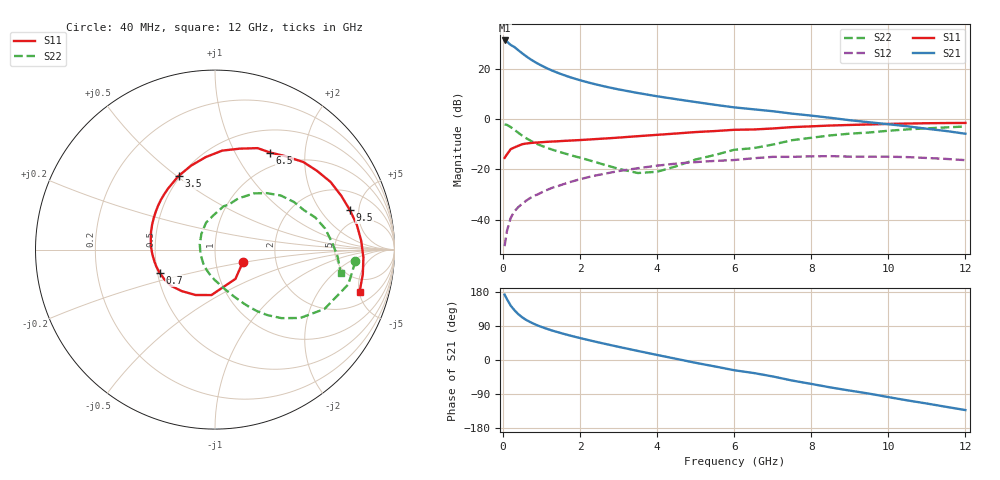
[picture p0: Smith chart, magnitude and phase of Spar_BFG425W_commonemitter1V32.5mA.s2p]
! Filename: 132bfg425.001
! BFG425W Field C1
! V1=8.907E-001V,V2=1.000E+000V, I1=5.288E-004A, I2=3.253E-002A
# GHz  S  MA  R 50
!  S11  S21  S12  S22
!Freq(GHz)  Mag  Ang  Mag  Ang  Mag  Ang  Mag  Ang
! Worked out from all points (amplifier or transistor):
!   44 points, 40 MHz to 12 GHz, reference 50 ohm
!   highest |S21| = 31.2 dB at 40 MHz (marker M1)
!   |S21| within 3 dB of that: start of sweep to 325.7 MHz
!   unconditionally stable (mu >= 1): start of sweep to 94.4 MHz; 717.5 MHz to end of sweep
!   at 700 MHz: K = 0.99, MSG = 27.6 dB, |S12| = -31.4 dB
!   at 2.4 GHz: K = 1.26, MAG = 15.1 dB, |S12| = -22.4 dB
!   at 12 GHz: K = 1.43, MAG = 1.3 dB, |S12| = -16.3 dB
!   S11 on the Smith chart (normalised r, x): 40 MHz: 1.35, -0.20; 700 MHz: 0.51, -0.15; 3.5 GHz: 0.49, +0.51; 6.5 GHz: 0.79, +1.40; 9.5 GHz: 3.51, +3.99; 12 GHz: 3.21, -5.06
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0.04  0.17 -24.8  36.42 172.5  0.003 72.4  0.785 -4.8
0.1  0.199 -55.0  34.55 160.7  0.006 78.8  0.768 -14.6
0.2  0.254 -94.5  29.6 143.1  0.011 70.9  0.694 -28.4
0.3  0.275 -113.0  26.76 130.8  0.015 67.2  0.609 -38.7
0.4  0.296 -128.5  23.16 120.5  0.018 64.2  0.532 -45.9
0.5  0.318 -140.7  20.13 112.3  0.021 62.4  0.468 -51.3
0.6  0.327 -149.7  17.66 105.8  0.024 61.6  0.418 -55.4
0.7  0.334 -157.1  15.63 100.3  0.027 60.8  0.377 -58.8
0.8  0.34 -163.4  14 95.4  0.03 60.3  0.344 -61.6
0.9  0.344 -168.8  12.66 91.1  0.032 59.8  0.317 -64.0
1.2  0.356 178.1  9.728 80.2  0.041 57.6  0.259 -70.9
1.4  0.362 170.9  8.405 74.0  0.046 55.9  0.231 -75.2
1.7  0.373 161.2  6.95 65.6  0.055 52.8  0.198 -82.0
2.2  0.392 147.3  5.362 53.0  0.07 46.7  0.155 -95.8
2.8  0.419 132.3  4.178 39.2  0.087 38.3  0.114 -118.5
3.5  0.458 116.3  3.293 23.9  0.106 27.6  0.085 -161.2
4.5  0.518 95.7  2.483 3.0  0.131 11.5  0.116 130.8
6.5  0.622 60.4  1.565 -34.3  0.167 -18.0  0.265 72.5
8.5  0.746 30.4  1.06 -72.4  0.184 -53.7  0.475 39.4
9.5  0.783 16.3  0.866 -88.7  0.179 -69.3  0.542 23.9
10.5  0.816 3.5  0.718 -106.7  0.176 -86.5  0.625 10.8
12  0.839 -16.2  0.512 -132.2  0.153 -113.8  0.713 -10.5
